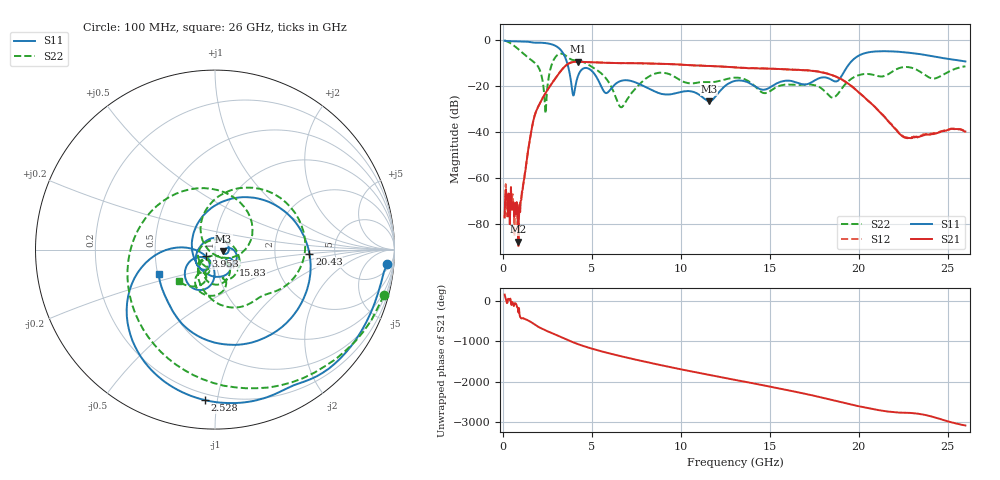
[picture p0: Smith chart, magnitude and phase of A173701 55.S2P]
!  2-Port S-parameters saved by WinCal
! VAR MeasName=S-Parameters (CALIBRATED_DATA) read from VNA (N5245A)
! VAR MeasDate=2017-6-7 10:32:02
! VAR NAME=A173701 55
! VAR FILENAME=A173701 55.S2P
! VAR DATE=2017-6-7 10:32:02
! VAR PHYS_PORTS=1,2
# Hz S DB R 50
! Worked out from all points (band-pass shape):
!   801 points, 100 MHz to 26 GHz, reference 50 ohm
!   highest |S21| = -9.44 dB at 4.212 GHz (marker M1); lowest = -87.6 dB at 877 MHz (marker M2)
!   |S21| within 3 dB of the highest: 3.369 GHz to 14.82 GHz (11.45 GHz wide, 126 % of centre)
!   lowest |S11| = -26.6 dB at 11.59 GHz (marker M3), VSWR 1.10, Z = 54.8 - j1.11 ohm
!   |S11| at or under -10 dB: 3.617 GHz to 19.51 GHz (15.9 GHz wide, 137 % of centre)
!   |S22| runs from -31.9 to -0.2 dB; largest |S21 - S12| = 0.0035
!   S11 on the Smith chart (normalised r, x): 100 MHz: 9, -20; 2.528 GHz: 0.16, -0.92; 3.953 GHz: 0.90, -0.07; 15.83 GHz: 1.20, -0.20; 20.43 GHz: 3.21, -0.21; 26 GHz: 0.51, -0.16
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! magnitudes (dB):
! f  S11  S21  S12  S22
! 100 MHz  -0.3  -77.0  -77.3  -0.2
! 877 MHz  -0.6  -87.6  -89.5  -4.0
! 1.719 GHz  -1.1  -34.9  -34.9  -9.4
! 2.366 GHz  -1.3  -23.5  -23.5  -28.5
! 2.528 GHz  -1.5  -21.5  -21.5  -18.9
! 3.014 GHz  -2.8  -16.0  -16.0  -6.9
! 3.953 GHz  -24.1  -9.6  -9.6  -8.7
! 4.212 GHz  -15.9  -9.4  -9.4  -8.9
! 4.438 GHz  -12.8  -9.5  -9.5  -9.3
! 5.798 GHz  -23.1  -10.0  -9.9  -16.7
! 6.64 GHz  -17.8  -10.1  -10.0  -29.2
! 8.744 GHz  -23.0  -10.3  -10.3  -14.3
! 11.59 GHz  -26.6  -11.3  -11.3  -18.3
! 13.05 GHz  -17.8  -11.9  -11.9  -16.4
! 15.83 GHz  -17.8  -12.7  -12.7  -19.4
! 17.39 GHz  -18.2  -13.4  -13.3  -19.4
! 18.59 GHz  -17.8  -15.5  -15.5  -25.0
! 20.43 GHz  -5.6  -25.7  -25.7  -14.7
! 21.69 GHz  -4.9  -35.6  -35.5  -14.7
! 22.73 GHz  -5.5  -42.7  -42.4  -11.7
! 24.22 GHz  -7.1  -40.6  -40.4  -16.8
! 26 GHz  -9.3  -39.8  -39.7  -11.5
